(* Logix 5000 AddOnInstructionDefinition export AMP_Normal_Stop; software revision 20.04 *)

TYPE AMP_Status_Word :   // Applied Motion Input Assembly Status Word
STRUCT
   Enabled : BOOL;   // Motor Enabled (Motor Disabled if this bit = 0)
   Sampling : BOOL;   // Sampling (for Quick Tuner)
   Drive_Fault : BOOL;   // Drive Fault (check Alarm Code)
   In_Position : BOOL;   // In Position (motor is in position)
   Moving : BOOL;   // Moving (motor is moving)
   Jogging : BOOL;   // Jogging (currently in jog mode)
   Stopping : BOOL;   // Stopping (in the process of stopping from a stop command)
   Waiting : BOOL;   // Waiting (for an input; executing a WI command)
   Saving : BOOL;   // Saving (parameter data is being saved)
   Alarm_Present : BOOL;   // Alarm present (check Alarm Code)
   Homing : BOOL;   // Homing (executing an SH command)
   Wait_Time : BOOL;   // Waiting (for time; executing a WD or WT command)
   Wizard_Running : BOOL;   // Wizard running (Timing Wizard is running)
   Checking_Encoder : BOOL;   // Checking encoder (Timing Wizard is running)
   Q_Program_Running : BOOL;   // Q Program is running
   Initializing : BOOL;   // Initializing (happens at power up) ; Servo Ready (for SV200 drives only)
END_STRUCT
END_TYPE

TYPE AMP_Input_Assembly_v2 :   // Applied Motion Drive Input Assembly Version 2.0
STRUCT
   Status_Code : DINT;   // Status Code
   Alarm_Code : DINT;   // Alarm Code
   Voltage : DINT;   // Supply Voltage (x0.1V)
   Current : DINT;   // Actual Current (mA)
   Temp : DINT;   // Drive Temperature (0.1 deg C)
   Encoder_Position : DINT;   // Encoder Position (20,000 counts = 1 shaft turn)
   Absolute_Position : DINT;   // Absolute Position (20,000 counts = 1 shaft turn)
   Position_Error : DINT;   // Position Error (counts)
   Actual_Velocity : DINT;   // Actual Velocity (rev/sec * 240, 0 when no encoder)
   Extended_Inputs : DINT;   // Input Status (Extended)
   Main_Board_Inputs : DINT;   // Input Status (Main board)
   Word11 : DINT;   // Reserved
   Analog_Input_1 : DINT;   // Analog Input 1 (ADC counts, 0=min V, 16383 = max V)
   Analog_Input_2 : DINT;   // Analog Input 2 (ADC counts, 0=min V, 16383 = max V)
END_STRUCT
END_TYPE

ADD_ON_INSTRUCTION AMP_Normal_Stop   (* revision 1.0 *)
// Applied Motion - Stop/Kill using Normal Deceleration - AOI
// Help:
// The Normal Stop AOI is used to stop and kill the drive using the normal deceleration set by the DE command.
VAR_IN_OUT
   Input : DINT[14]; {required}   // Drive Input Assembly
   Output : DINT[16]; {required}   // Drive Output Assembly
        [0]   // Command Word
        [1]   // Jog Speed (0.25 rev/min)
        [2]   // Jog Acceleration (10 rev/s/s)
        [3]   // Jog Deceleration (10 rev/s/s)
        [4]   // Point-to-Point Velocity (0.25 rev/min)
        [5]   // Point-to-Point Acceleration (10 rev/s/s)
        [6]   // Point-to-Point Deceleration (10 rev/s/s)
        [7]   // Point-to-Point Distance (Motor steps)
        [9]   // (2x ASCII Letters in 16 lower word)
        [10]   // Data/Register 1
        [11]   // Data/Register 2
END_VAR
VAR_INPUT
   RPI : DINT := 100; {visible}   // Drive Connection Request Packet Interval (milliseconds)
   Stop : BOOL; {required}   // Stop the drive axis
END_VAR
VAR_OUTPUT
   Sent : BOOL; {access Read Only, visible}   // Stop has been sent to drive
   In_Progress : BOOL; {access Read Only, visible}   // Stop in progress
   Done : BOOL; {access Read Only, visible}   // Stop completed without errors - Servo is not moving
   Error : BOOL; {access Read Only, visible}   // Stop failed - drive not ready or faulted
   State : DINT := 10; {access None}   // Internal state of progress
END_VAR
VAR
   Loc_StatusCode : AMP_Status_Word;
   Loc_CommandOff_Timer : TIMER;   // Timer to make sure command value was 0 before sending a new command
   Loc_CommandOn_Timer : TIMER;   // Timer to make sure command value is set long enough to be sent to servo
   Loc_Input_Assembly : AMP_Input_Assembly_v2; {access None}
   Loc_Stop_ONS : BOOL; {access None}
END_VAR

ROUTINE Logic   (* ladder *)
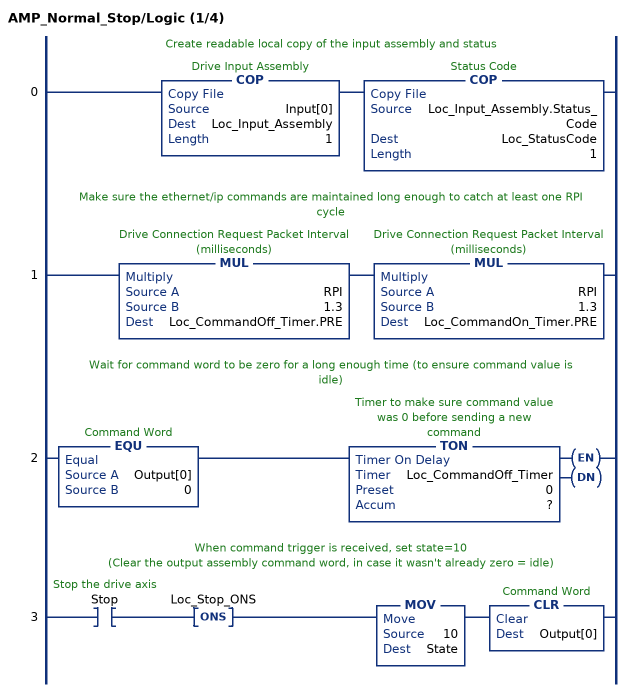
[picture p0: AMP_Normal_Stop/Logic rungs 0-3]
   // Create readable local copy of the input assembly and status
   0: COP(Input[0],Loc_Input_Assembly,1)COP(Loc_Input_Assembly.Status_Code,Loc_StatusCode,1);
   // Make sure the ethernet/ip commands are maintained long enough to catch at least one RPI cycle
   1: MUL(RPI,1.3,Loc_CommandOff_Timer.PRE)MUL(RPI,1.3,Loc_CommandOn_Timer.PRE);
   // Wait for command word to be zero for a long enough time (to ensure command value is idle)
   2: EQU(Output[0],0)TON(Loc_CommandOff_Timer,?,?);
   // When command trigger is received, set state=10
   // (Clear the output assembly command word, in case it wasn't already zero = idle)
   3: XIC(Stop)ONS(Loc_Stop_ONS)MOV(10,State)CLR(Output[0]);
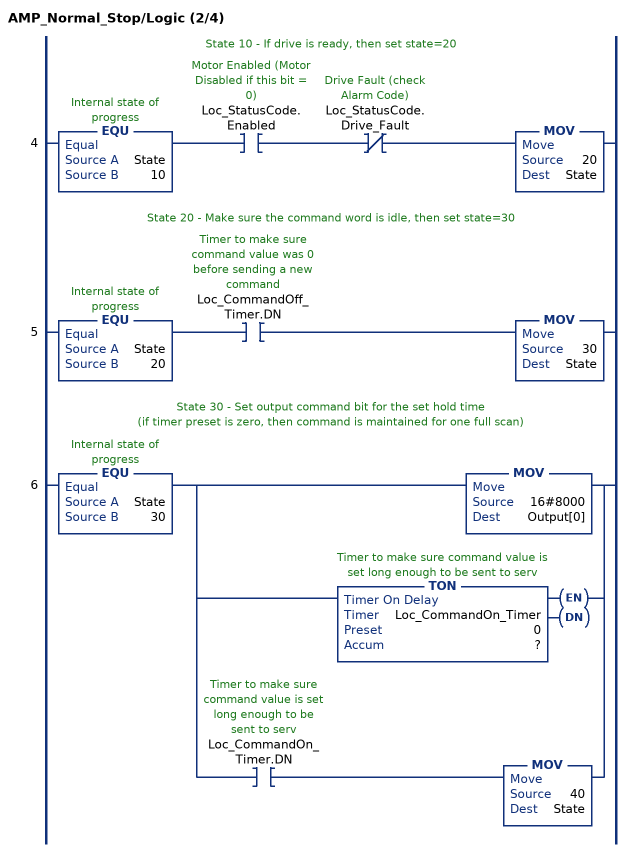
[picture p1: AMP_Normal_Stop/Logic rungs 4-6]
   // State 10 - If drive is ready, then set state=20
   4: EQU(State,10)XIC(Loc_StatusCode.Enabled)XIO(Loc_StatusCode.Drive_Fault)MOV(20,State);
   // State 20 - Make sure the command word is idle, then set state=30
   5: EQU(State,20)XIC(Loc_CommandOff_Timer.DN)MOV(30,State);
   // State 30 - Set output command bit for the set hold time
   // (if timer preset is zero, then command is maintained for one full scan)
   6: EQU(State,30)[MOV(16#8000,Output[0]) ,TON(Loc_CommandOn_Timer,?,?) ,XIC(Loc_CommandOn_Timer.DN) MOV(40,State) ];
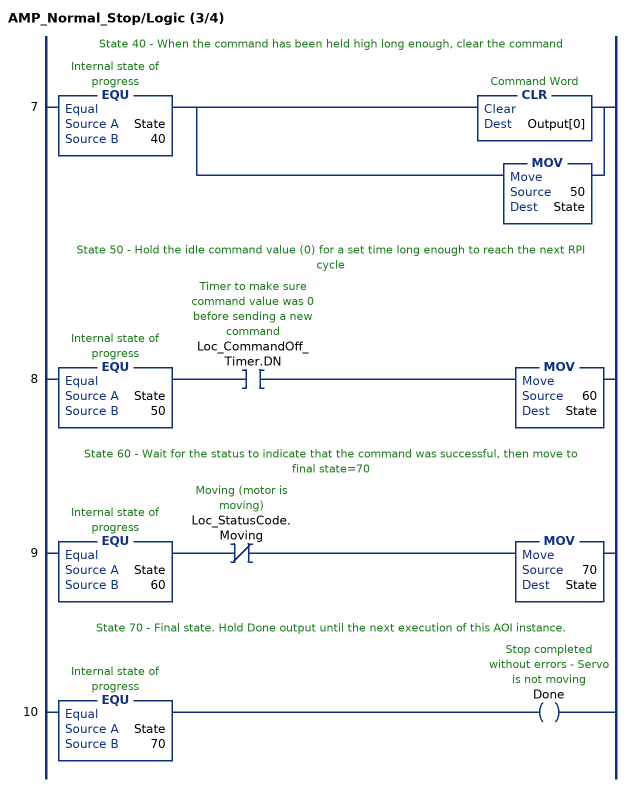
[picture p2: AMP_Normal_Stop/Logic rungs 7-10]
   // State 40 - When the command has been held high long enough, clear the command
   7: EQU(State,40)[CLR(Output[0]) ,MOV(50,State) ];
   // State 50 - Hold the idle command value (0) for a set time long enough to reach the next RPI cycle
   8: EQU(State,50)XIC(Loc_CommandOff_Timer.DN)MOV(60,State);
   // State 60 - Wait for the status to indicate that the command was successful, then move to final state=70
   9: EQU(State,60)XIO(Loc_StatusCode.Moving)MOV(70,State);
   // State 70 - Final state. Hold Done output until the next execution of this AOI instance.
   10: EQU(State,70)OTE(Done);
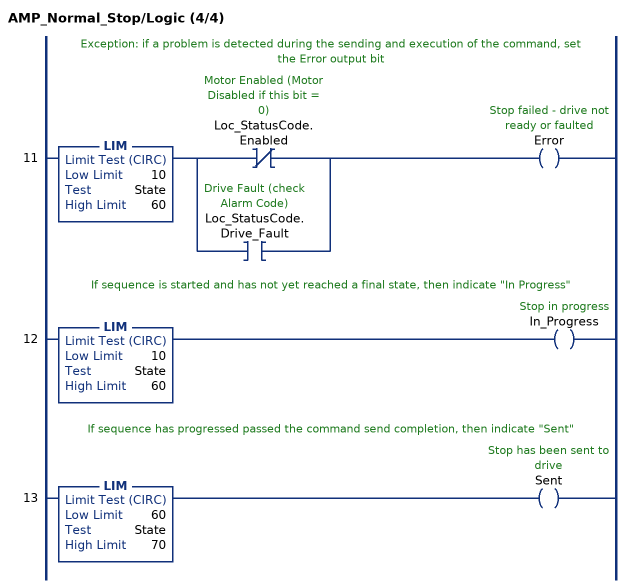
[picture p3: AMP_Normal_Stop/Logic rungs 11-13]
   // Exception: if a problem is detected during the sending and execution of the command, set the Error output bit
   11: LIM(10,State,60)[XIO(Loc_StatusCode.Enabled) ,XIC(Loc_StatusCode.Drive_Fault) ]OTE(Error);
   // If sequence is started and has not yet reached a final state, then indicate "In Progress"
   12: LIM(10,State,60)OTE(In_Progress);
   // If sequence has progressed passed the command send completion, then indicate "Sent"
   13: LIM(60,State,70)OTE(Sent);
END_ROUTINE
END_ADD_ON_INSTRUCTION
